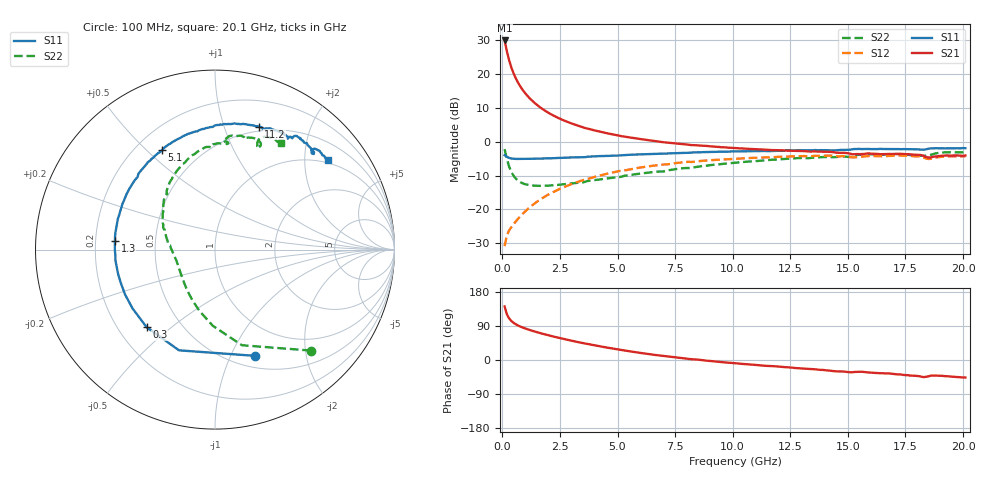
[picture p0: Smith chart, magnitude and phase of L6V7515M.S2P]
!  Infineon Technologies AG
! BFR380L3 , PF131585-7, No.6, Th 09.10.01, soldered on pcb-board, measured with PP GSG850
!  Vce=0.75 V,  Ic=15.0 mA
! Common Emitter S-Parameters:  15. November 2001
#  GHz  S  MA  R  50
! f  S11  S21  S12  S22
! GHz  Mag  Ang  Mag  Ang  Mag  Ang  Mag  Ang
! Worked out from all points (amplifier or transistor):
!   201 points, 100 MHz to 20.1 GHz, reference 50 ohm
!   highest |S21| = 29.8 dB at 100 MHz (marker M1)
!   |S21| within 3 dB of that: start of sweep to 192.5 MHz
!   unconditionally stable (mu >= 1): 1.448 GHz to 5.273 GHz; 18.37635 GHz to 18.44061 GHz
!   at 3.4 GHz: K = 1.03, MAG = 6.9 dB, |S12| = -11.6 dB
!   at 10.1 GHz: K = 0.98, MSG = 1.6 dB, |S12| = -5.0 dB
!   at 20.1 GHz: K = 0.99, MSG = 0.1 dB, |S12| = -4.3 dB
!   S11 on the Smith chart (normalised r, x): 100 MHz: 0.63, -1.24; 300 MHz: 0.32, -0.41; 1.3 GHz: 0.28, +0.04; 5.1 GHz: 0.31, +0.56; 11.2 GHz: 0.45, +1.31; 20.1 GHz: 0.93, +2.58
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0.1  0.6316 -69.5  31.06 141.3  0.02879 61.2  0.7762 -46.5
0.2  0.5959 -109.6  21.38 120.3  0.04174 50.5  0.5536 -74.2
0.3  0.5762 -131.4  15.66 109.4  0.0495 48.4  0.4256 -91.5
0.4  0.5644 -144.4  12.2 102.5  0.05537 49.2  0.3533 -104.1
0.5  0.5601 -153.6  9.953 97.5  0.06129 50.8  0.31 -113.8
0.6  0.5566 -160.4  8.377 93.8  0.06767 52.7  0.2824 -121.6
0.7  0.5568 -165.7  7.247 90.5  0.07389 54.2  0.2638 -128.2
0.8  0.5557 -169.9  6.375 87.8  0.08067 55.5  0.2509 -133.7
0.9  0.5579 -173.6  5.693 85.3  0.08745 56.6  0.2419 -138.5
1  0.5561 -176.9  5.148 83.1  0.0942 57.5  0.2356 -142.6
1.3  0.5595 175.0  4.005 77.0  0.1153 59.0  0.2259 -152.3
1.7  0.5642 166.3  3.104 70.0  0.1443 59.2  0.2236 -161.5
2.1  0.5689 158.9  2.551 63.8  0.1732 58.3  0.2265 -168.3
2.7  0.5798 149.1  2.036 55.0  0.2158 55.7  0.2367 -176.8
3.5  0.591 137.5  1.629 44.5  0.2709 51.0  0.2512 174.7
5.1  0.6274 118.1  1.222 26.7  0.3699 40.0  0.3013 158.3
6.8  0.6647 101.0  1.003 12.0  0.4534 28.4  0.3628 141.6
10.1  0.7181 76.8  0.8047 -8.6  0.5602 7.3  0.4891 115.5
11.2  0.7273 70.5  0.7675 -14.1  0.5836 0.6  0.5237 107.2
13.5  0.7481 59.5  0.719 -24.3  0.6144 -12.4  0.5808 91.6
16.8  0.777 47.7  0.6605 -35.5  0.616 -27.3  0.6531 72.9
20.1  0.8017 38.4  0.6265 -46.2  0.6093 -40.4  0.6994 58.1
